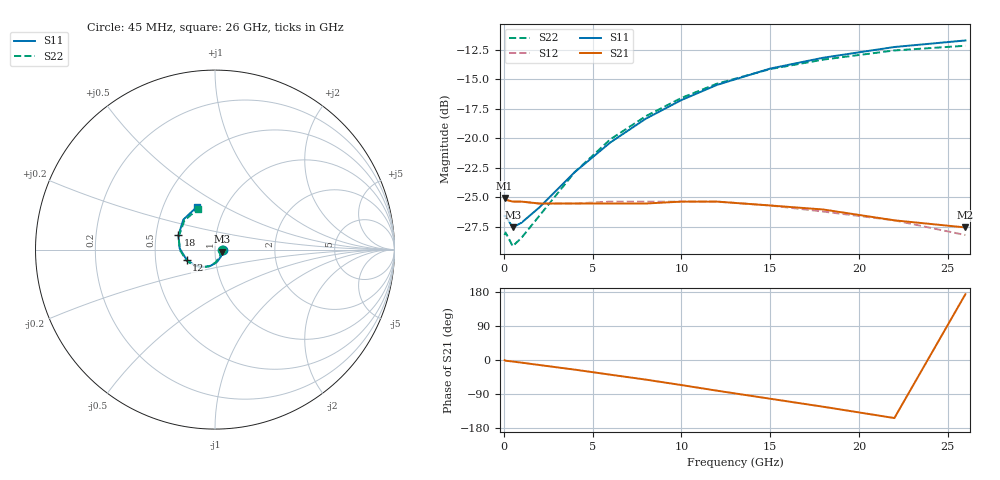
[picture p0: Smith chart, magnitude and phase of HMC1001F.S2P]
! HMMC-1001
! Typical s-parameters at 25dB attenuation setting , TA = 25 C
# ghz s ma r 50
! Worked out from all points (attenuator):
!   14 points, 45 MHz to 26 GHz, reference 50 ohm
!   highest |S21| = -25.04 dB at 45 MHz (marker M1); lowest = -27.5 dB at 26 GHz (marker M2)
!   lowest |S11| = -27.5 dB at 500 MHz (marker M3), VSWR 1.09, Z = 54.2 - j1.2 ohm
!   |S11| at or under -10 dB: start of sweep to end of sweep
!   |S22| runs from -29.1 to -12.2 dB; largest |S21 - S12| = 0.0032
!   S11 on the Smith chart (normalised r, x): 45 MHz: 1.10, -0.00; 12 GHz: 0.72, -0.08; 18 GHz: 0.65, +0.11; 26 GHz: 0.74, +0.38
0.045  0.047 -2.1  0.056 -0.5  0.056 -0.5  0.039 -3.1
0.1  0.047 -5.1  0.055 -1.9  0.055 -1.6  0.04 -7.1
0.5  0.042 -15.3  0.054 -4.0  0.054 -3.7  0.035 -18.2
1  0.044 -27.1  0.054 -7.0  0.054 -6.8  0.038 -32.1
2  0.051 -49.1  0.053 -13.2  0.053 -13.2  0.047 -56.1
4  0.072 -82.8  0.053 -25.5  0.053 -25.7  0.072 -88.0
6  0.096 -106.9  0.053 -38.7  0.054 -38.5  0.099 -109.4
8  0.121 -126.4  0.053 -51.8  0.054 -51.9  0.124 -127.5
10  0.145 -144.3  0.054 -66.1  0.054 -66.2  0.148 -143.6
12  0.168 -160.4  0.054 -80.9  0.054 -81.0  0.17 -158.7
15  0.197 178.0  0.052 -102.2  0.052 -103.3  0.196 -179.5
18  0.219 158.6  0.05 -123.4  0.049 -124.1  0.215 160.3
22  0.243 136.4  0.045 -153.2  0.045 -154.1  0.235 136.6
26  0.259 112.6  0.042 173.6  0.039 175.0  0.246 112.8
